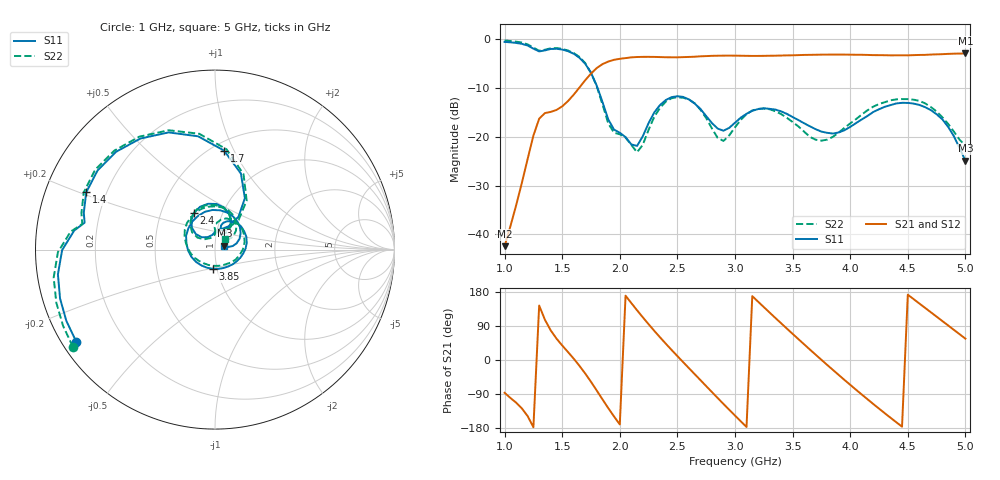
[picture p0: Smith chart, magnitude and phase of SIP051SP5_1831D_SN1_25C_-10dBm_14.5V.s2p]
# GHz  S  dB  R  50
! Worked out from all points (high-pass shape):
!   81 points, 1 GHz to 5 GHz, reference 50 ohm
!   highest |S21| = -3.02 dB at 5 GHz (marker M1); lowest = -42.4 dB at 1 GHz (marker M2)
!   |S21| within 3 dB of the highest: 1.799 GHz to end of sweep
!   lowest |S11| = -24.9 dB at 5 GHz (marker M3), VSWR 1.12, Z = 55.5 + j2.35 ohm
!   |S11| at or under -10 dB: 1.806 GHz to end of sweep
!   |S22| runs from -23.2 to -0.4 dB; largest |S21 - S12| = 0.0022
!   S11 on the Smith chart (normalised r, x): 1 GHz: 0.04, -0.30; 1.4 GHz: 0.13, +0.21; 1.7 GHz: 0.57, +0.91; 2.4 GHz: 0.73, +0.32; 3.85 GHz: 0.95, -0.21; 5 GHz: 1.11, +0.05
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1  -0.65 -146.4  -42.39 -86.6  -42.30 -89.3  -0.36 -145.6
1.3  -2.60 168.4  -16.35 143.7  -16.34 143.8  -2.46 169.1
1.4  -2.10 156.0  -14.96 78.3  -14.97 78.2  -1.96 156.4
1.55  -2.55 123.9  -12.75 21.1  -12.74 21.2  -2.41 123.9
1.7  -5.13 84.8  -8.48 -35.8  -8.49 -35.7  -4.99 83.5
1.85  -12.97 54.4  -5.19 -104.1  -5.19 -104.2  -13.45 51.5
2.05  -20.12 89.8  -3.97 169.8  -3.96 169.8  -20.20 87.5
2.2  -19.91 137.0  -3.71 112.5  -3.71 112.5  -21.66 136.0
2.35  -13.53 128.8  -3.76 59.5  -3.76 59.6  -14.10 134.8
2.4  -12.53 119.4  -3.79 42.8  -3.79 42.8  -12.84 124.6
2.55  -11.90 87.9  -3.77 -5.7  -3.78 -5.6  -12.07 90.5
2.75  -15.81 57.6  -3.56 -69.0  -3.55 -68.9  -16.23 55.5
3  -17.17 76.1  -3.46 -146.7  -3.46 -146.7  -18.10 90.9
3.2  -14.38 51.2  -3.52 154.0  -3.52 154.1  -14.35 60.2
3.4  -14.85 12.3  -3.44 97.1  -3.43 97.1  -15.40 14.0
3.7  -18.49 -52.8  -3.28 14.0  -3.27 14.1  -20.64 -77.1
3.85  -19.38 -96.8  -3.24 -26.1  -3.24 -26.1  -20.05 -130.2
4.1  -16.51 -177.5  -3.29 -90.9  -3.29 -91.0  -15.50 166.2
4.35  -13.57 116.9  -3.40 -152.4  -3.39 -152.3  -12.59 117.0
4.55  -13.26 71.9  -3.36 160.8  -3.36 160.7  -12.46 79.4
4.75  -15.43 32.6  -3.20 114.4  -3.20 114.4  -14.88 48.6
5  -24.93 21.8  -3.02 56.3  -3.02 56.4  -21.81 46.9
